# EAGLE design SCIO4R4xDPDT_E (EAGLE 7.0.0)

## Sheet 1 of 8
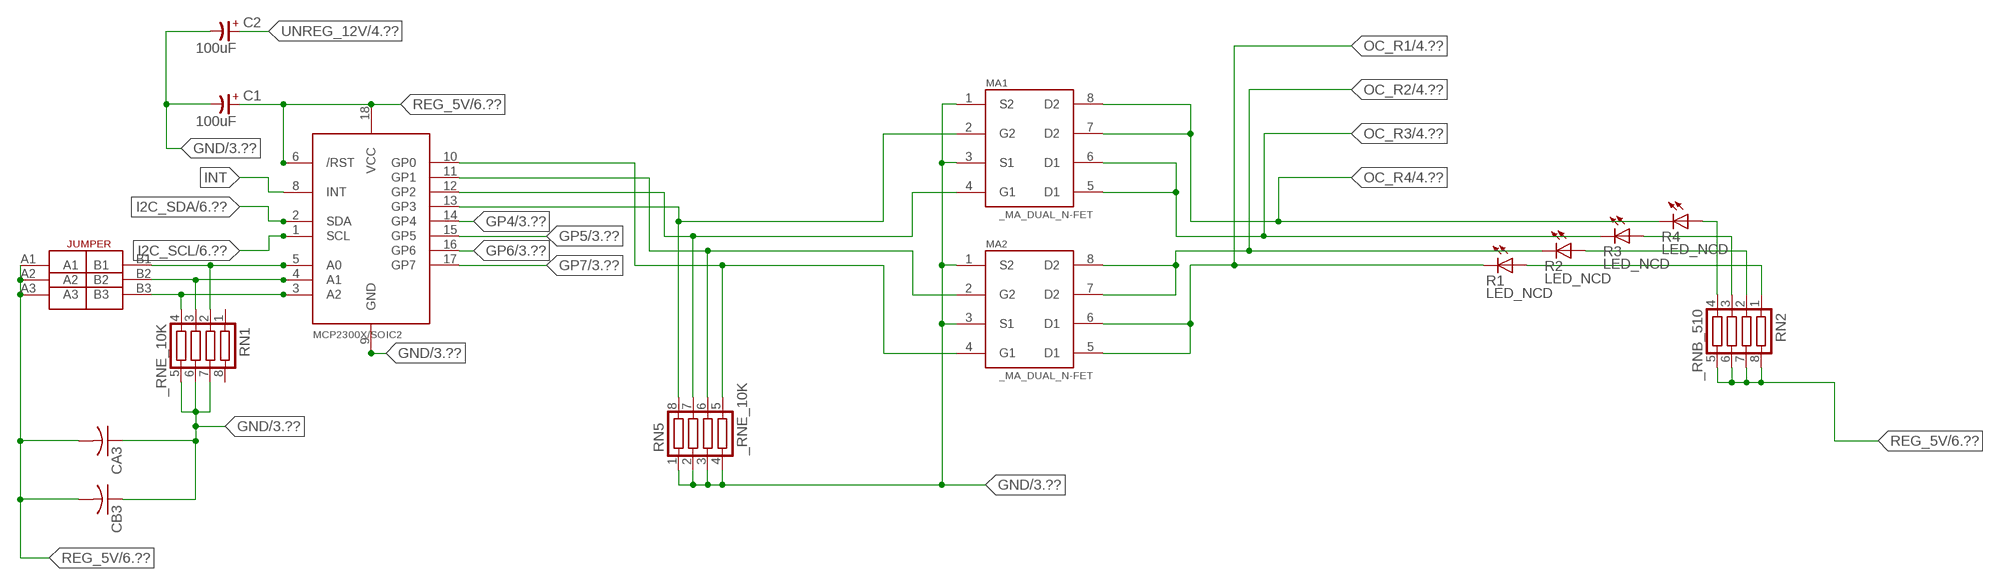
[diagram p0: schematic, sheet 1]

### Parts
C1  100uF  CP-E-025X060  [E-025X060]
C2  100uF  CP-E-025X060  [E-025X060]
CA3  CC1206KRX7R9BB104C1206K  [CC1206KRX7R9BB104]
CB3  TMK316F106ZL-TC1206K  [TMK316F106ZL-T]
IC2  MCP2300X/SO  [SO18W]
MA1  _MA_DUAL_N-FET  [_MA_DUAL_N-FET]
MA2  _MA_DUAL_N-FET  [_MA_DUAL_N-FET]
R1  LED_NCD  [CHIPLED_0603]
R2  LED_NCD  [CHIPLED_0603]
R3  LED_NCD  [CHIPLED_0603]
R4  LED_NCD  [CHIPLED_0603]
RN1  _RNE_10K  [RNE]
RN2  _RNB_510  [RNB]
RN5  _RNE_10K  [RNE]
U$18  JUMPER_3X2  [JUMPER_3X2]

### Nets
GND: C1.- C2.- CA3.1 CB3.1 IC2.9(GND) MA1.1(S2) MA1.3(S1) MA2.1(S2) MA2.3(S1) RN1.5 RN1.6 RN1.7 RN5.1 RN5.2 RN5.3 RN5.4 ; also sheet 3,6,8
GP4: IC2.14(GP4) ; also sheet 3
GP5: IC2.15(GP5) ; also sheet 3
GP6: IC2.16(GP6) ; also sheet 3
GP7: IC2.17(GP7) ; also sheet 3
I2C_SCL: IC2.1(SCL) ; also sheet 6
I2C_SDA: IC2.2(SDA) ; also sheet 6
INT: IC2.8(INT)
N$6: IC2.5(A0) RN1.2 U$18.B1
N$7: IC2.4(A1) RN1.3 U$18.B2
N$8: IC2.3(A2) RN1.4 U$18.B3
N$20: IC2.13(GP3) MA1.2(G2) RN5.8
N$21: IC2.12(GP2) MA1.4(G1) RN5.7
N$22: IC2.11(GP1) MA2.2(G2) RN5.6
N$23: IC2.10(GP0) MA2.4(G1) RN5.5
N$29: R4.A RN2.4
N$30: R3.A RN2.3
N$31: R2.A RN2.2
N$32: R1.A RN2.1
OC_R1: MA2.5(D1) MA2.6(D1) R1.C ; also sheet 4
OC_R2: MA2.7(D2) MA2.8(D2) R2.C ; also sheet 4
OC_R3: MA1.5(D1) MA1.6(D1) R3.C ; also sheet 4
OC_R4: MA1.7(D2) MA1.8(D2) R4.C ; also sheet 4
REG_5V: C1.+ CA3.2 CB3.2 IC2.6(/RST) IC2.18(VCC) RN2.5 RN2.6 RN2.7 RN2.8 U$18.A1 U$18.A2 U$18.A3 ; also sheet 6,8
UNREG_12V: C2.+ ; also sheet 4,6
Unconnected: RN1.1 RN1.8

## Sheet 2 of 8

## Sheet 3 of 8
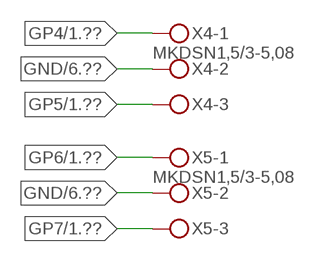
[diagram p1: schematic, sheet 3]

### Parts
X4  MKDSN1,5/3-5,08  [MKDSN1,5/3-5,08]
X5  MKDSN1,5/3-5,08  [MKDSN1,5/3-5,08]

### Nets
GND: X4.2 X5.2 ; also sheet 1,6,8
GP4: X4.1 ; also sheet 1
GP5: X4.3 ; also sheet 1
GP6: X5.1 ; also sheet 1
GP7: X5.3 ; also sheet 1

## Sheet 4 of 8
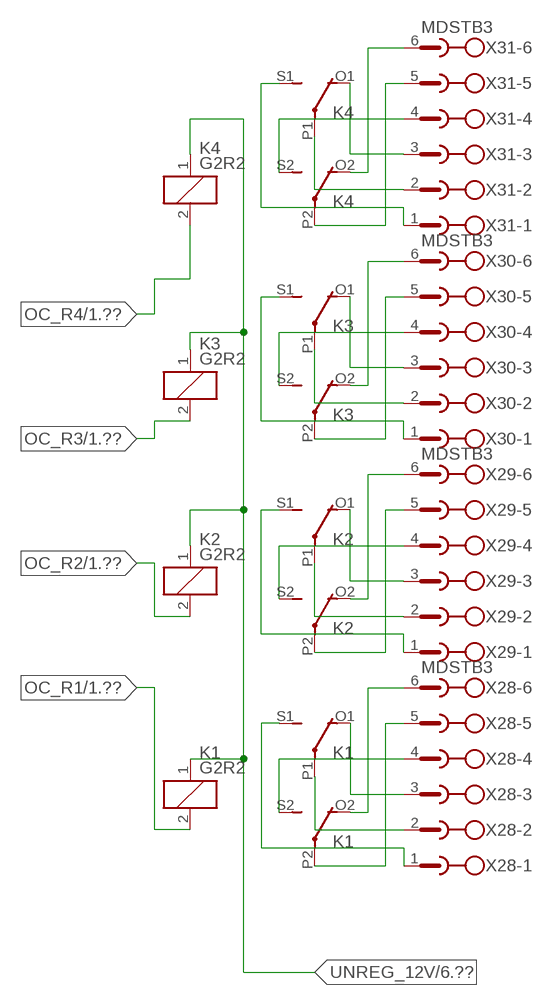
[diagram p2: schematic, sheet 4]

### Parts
K1  G2R2  [G2R2]
K2  G2R2  [G2R2]
K3  G2R2  [G2R2]
K4  G2R2  [G2R2]
X28  MDSTB3  [MDSTB3]
X29  MDSTB3  [MDSTB3]
X30  MDSTB3  [MDSTB3]
X31  MDSTB3  [MDSTB3]

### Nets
N$9: K3.P2(3:COM) X30.5
N$10: K3.O2(3:NC) X30.6
N$11: K4.P2(3:COM) X31.5
N$12: K4.O2(3:NC) X31.6
N$13: K3.S2(3:NO) X30.4
N$14: K4.S2(3:NO) X31.4
N$15: K3.O1(2:NC) X30.3
N$16: K4.O1(2:NC) X31.3
N$17: K4.P1(2:COM) X31.2
N$18: K3.P1(2:COM) X30.2
N$19: K3.S1(2:NO) X30.1
N$24: K4.S1(2:NO) X31.1
N$203: K1.P2(3:COM) X28.5
N$204: K1.O2(3:NC) X28.6
N$205: K1.S2(3:NO) X28.4
N$206: K1.P1(2:COM) X28.2
N$207: K1.O1(2:NC) X28.3
N$208: K1.S1(2:NO) X28.1
N$209: K2.P2(3:COM) X29.5
N$210: K2.O2(3:NC) X29.6
N$211: K2.S2(3:NO) X29.4
N$212: K2.S1(2:NO) X29.1
N$213: K2.P1(2:COM) X29.2
N$214: K2.O1(2:NC) X29.3
OC_R1: K1.2(1:C2) ; also sheet 1
OC_R2: K2.2(1:C2) ; also sheet 1
OC_R3: K3.2(1:C2) ; also sheet 1
OC_R4: K4.2(1:C2) ; also sheet 1
UNREG_12V: K1.1(1:C1) K2.1(1:C1) K3.1(1:C1) K4.1(1:C1) ; also sheet 1,6

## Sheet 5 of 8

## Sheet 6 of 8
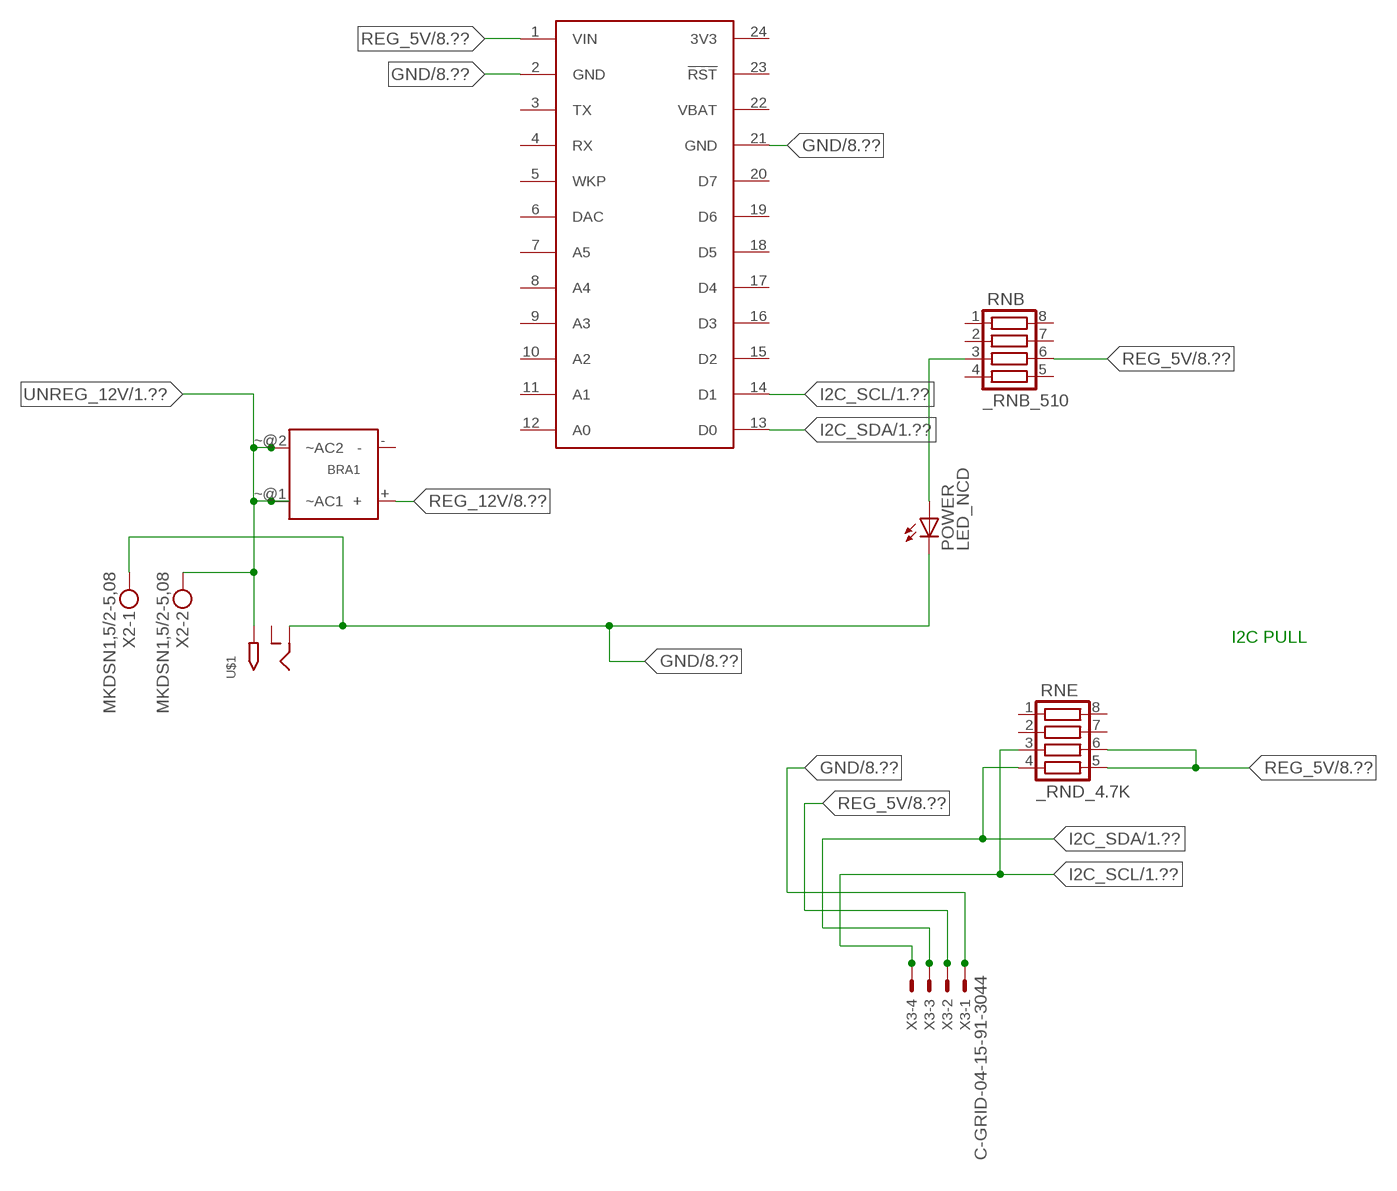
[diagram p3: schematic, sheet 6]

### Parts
BRA1  MB2S_  [MB2S]
POWER  LED_NCD  [CHIPLED_0603]
RNB  _RNB_510  [RNB]
RNE  _RND_4.7K  [RND]
S1  SPARK_CORECORE  [SPARK_CORE]
U$1  2.1MMJACK  [PJ-102A]
X2  MKDSN1,5/2-5,08  [MKDSN1,5/2-5,08]
X3  C-GRID-04-15-91-3044  [15-91-04]

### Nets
GND: POWER.C S1.2(GND) S1.21(GND) U$1.RING X2.1 X3.1 ; also sheet 1,3,8
I2C_SCL: RNE.3 S1.14(D1) X3.4 ; also sheet 1
I2C_SDA: RNE.4 S1.13(D0) X3.3 ; also sheet 1
N$2: POWER.A RNB.3
REG_5V: RNB.6 RNE.5 RNE.6 S1.1(VIN) X3.2 ; also sheet 1,8
REG_12V: BRA1.+ ; also sheet 8
UNREG_12V: BRA1.~@1(~AC1) BRA1.~@2(~AC2) U$1.TIP X2.2 ; also sheet 1,4
Unconnected: BRA1.- RNB.1 RNB.2 RNB.4 RNB.5 RNB.7 RNB.8 RNE.1 RNE.2 RNE.7 RNE.8 S1.3(TX) S1.4(RX) S1.5(WKP) S1.6(DAC) S1.7(A5) S1.8(A4) S1.9(A3) S1.10(A2) S1.11(A1) S1.12(A0) S1.15(D2) S1.16(D3) S1.17(D4) S1.18(D5) S1.19(D6) S1.20(D7) S1.23(!RST) U$1.RING_SW

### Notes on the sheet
- I2C PULL

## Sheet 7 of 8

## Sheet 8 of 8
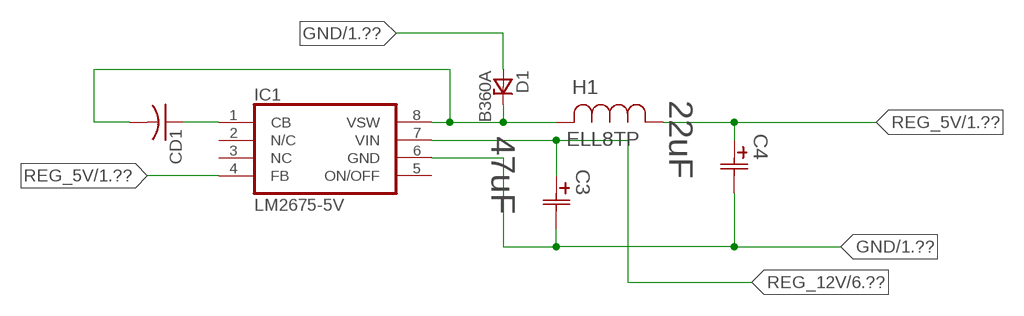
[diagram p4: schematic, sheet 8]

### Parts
C3  47uF  490-5463-6-NDCAP  [C2917(7343)-Y]
C4  22uF  490-5463-6-NDCAP  [C2917(7343)-Y]
CD1  _CD_10NF_50VC1206K  [_CD_10NF_50V]
D1  B360A  [DO214AC_ZENER]
H1  ELL8TP  [IND_ELL8TP]
IC1  LM2675-5V  LM2675  [SO-8]

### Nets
GND: C3.2(C2) C4.2(C2) D1.A IC1.6(GND) ; also sheet 1,3,6
N$1: CD1.2 D1.C H1.2 IC1.8(VSW)
N$3: CD1.1 IC1.1(CB)
REG_5V: C4.1(C1) H1.1 IC1.4(FB) ; also sheet 1,6
REG_12V: C3.1(C1) IC1.7(VIN) ; also sheet 6
Unconnected: IC1.2(N/C) IC1.5(ON/OFF)

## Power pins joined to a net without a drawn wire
3V3: S1.24(3V3)
NC: IC1.3(NC)
VBAT: S1.22(VBAT)

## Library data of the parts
BRA1 = NCD_ULTIMATE_LIBRARY:MB2S: Bridge Rectifier BRA MB2S 200V 500ma Digikey MB2S-TPMSTR-ND/MB2S-TP
C1 C2 = NCD_ULTIMATE_LIBRARY:CP-: Capacitors All Kinds POLARIZED CAP
C3 C4 = NCD_ULTIMATE_bhaskar:490-5463-6-ND: NCD CAP
CA3 = NCD_ULTIMATE_LIBRARY:CC1206KRX7R9BB104: Capacitor CA .1uF 50V SMT C1206K CC1206KRX7R9BB104
CB3 = NCD_ULTIMATE_LIBRARY:TMK316F106ZL-T: Capacitor CB 10uF SMT 1206 TMK316F106ZL-T
CD1 = NCD_ULTIMATE_LIBRARY:_CD_10NF_50V: Capacitor 10nF SMT
D1 = NCD_ULTIMATE_bhaskar:B360A: NCD DIODE B350A/B360A
H1 = NCD_ULTIMATE_bhaskar:ELL8TP: NCD coil
IC1 = NCD_ULTIMATE_bhaskar:LM2675: LM2675 NCD http://www.ti.com/lit/ds/symlink/lm2675.pdf
IC2 = NCD_ULTIMATE_LIBRARY:MCP2300X: Semiconductor Port Expander I/O 8-Bit I2C MCP23008 Inexpensive i2c i/o expander - 8 general purpose i/o pins with optional pullups
K1-K4 = NCD_ULTIMATE_LIBRARY:G2R2: RELAY 2 x switch, Omron
MA1 MA2 = NCD_ULTIMATE_LIBRARY:_MA_DUAL_N-FET: FET Dual N-Channel 8-SOIC NMOSFET Digikey 785-1064-2-ND/AO4842
POWER = NCD_ULTIMATE_bhaskar:LED_NCD
R1-R4 = NCD_ULTIMATE_LIBRARY:LED_NCD: LED Digikey 754-1132-2-ND/APT2012SRCPRV
RN1 RN5 = NCD_ULTIMATE_LIBRARY:_RNE_10K: Resistor Array RNE SMT 10K x 4 Single Resistor Source: http://www.ctscorp.com/components/Datasheets/CTSChipArrayDs.pdf Digikey 742C083103JPTR-ND/742C083103JP; OC_FARNELL: unknown; OC_NEWARK: unknown
RN2 RNB = NCD_ULTIMATE_LIBRARY:_RNB_510: Resistor Array RNB SMT 510 x 4 Single Resistor Source: http://www.ctscorp.com/components/Datasheets/CTSChipArrayDs.pdf Digikey 742C083511JPTR-ND/ 742C083511JP; OC_FARNELL: unknown; OC_NEWARK: unknown
RNE = NCD_ULTIMATE_LIBRARY:_RND_4.7K: Resistor Array RND SMT 4.7K x 4 Single Resistor Source: http://www.ctscorp.com/components/Datasheets/CTSChipArrayDs.pdf Digikey 742C083472JPTR-ND/742C083472JP; OC_FARNELL: unknown; OC_NEWARK: unknown
S1 = Spark:SPARK_CORE
U$1 = NCD_ULTIMATE_CONNECTORS:2.1MMJACK: 2.1mm x 5.5mm DC jack with internal switch. Digikey part #PJ-102A, 4UCON part #05537 By microbuilder.eu
U$18 = NCD_ULTIMATE_CONNECTORS:JUMPER_3X2
X2 = NCD_ULTIMATE_CONNECTORS:MKDSN1,5/2-5,08: MKDSN 1,5/ 2-5,08 Printklemme
X3 = NCD_ULTIMATE_CONNECTORS:C-GRID-04: CONNECTOR 4-Pos I2C wire to board 2.54 mm (0.100") pitch header Digikey WM1342-ND/0015912045; OC_FARNELL: unknown; OC_NEWARK: unknown
X4 X5 = NCD_ULTIMATE_CONNECTORS:MKDSN1,5/3-5,08: MKDSN 1,5/ 3-5,08 Printklemme Nennstrom: 13,5 A Nennspannung: 250 V Rastermaß: 5,08 mm Polzahl: 3 Anschlussart: Schraubanschluss Montage: Löten Anschlussrichtung Leiter/Platine: 0 ° Artikelnummer: 1729131 Source: http://eshop.phoenixcontact.com .. 1729131.pdf
X28-X31 = NCD_ULTIMATE_LIBRARY:MDSTB3: PHOENIX

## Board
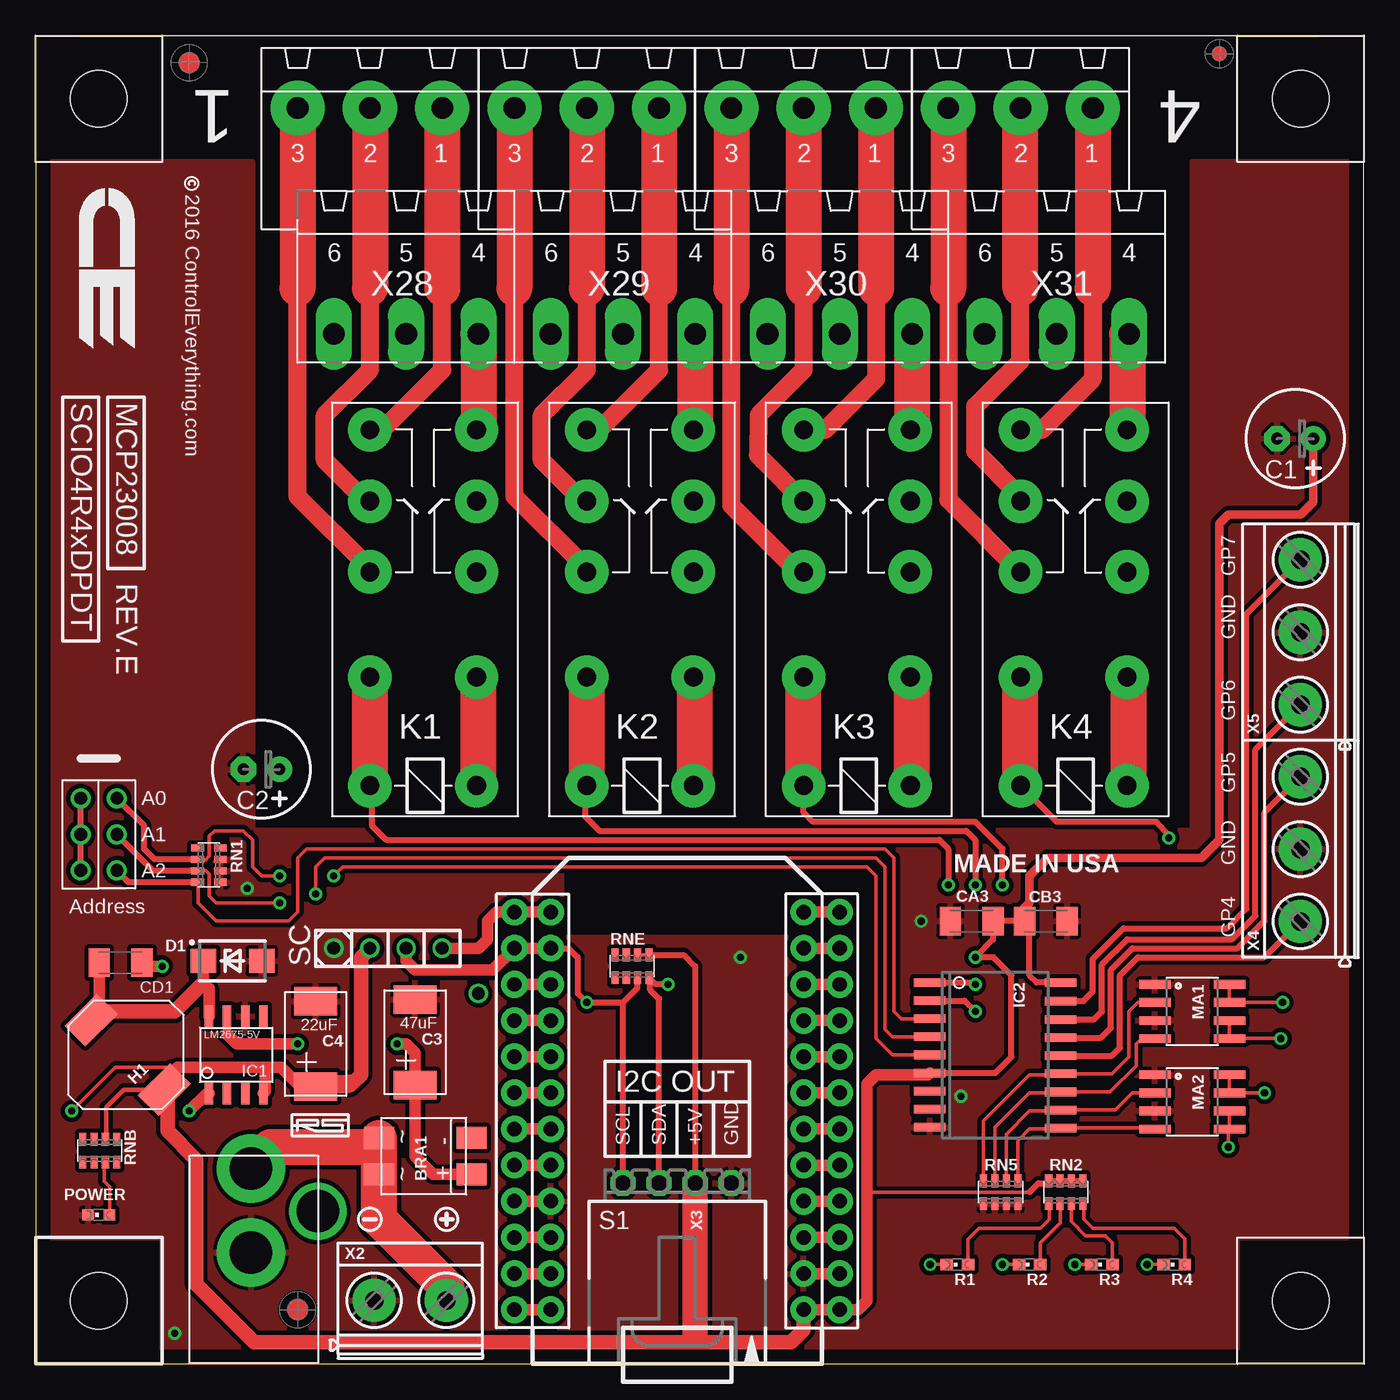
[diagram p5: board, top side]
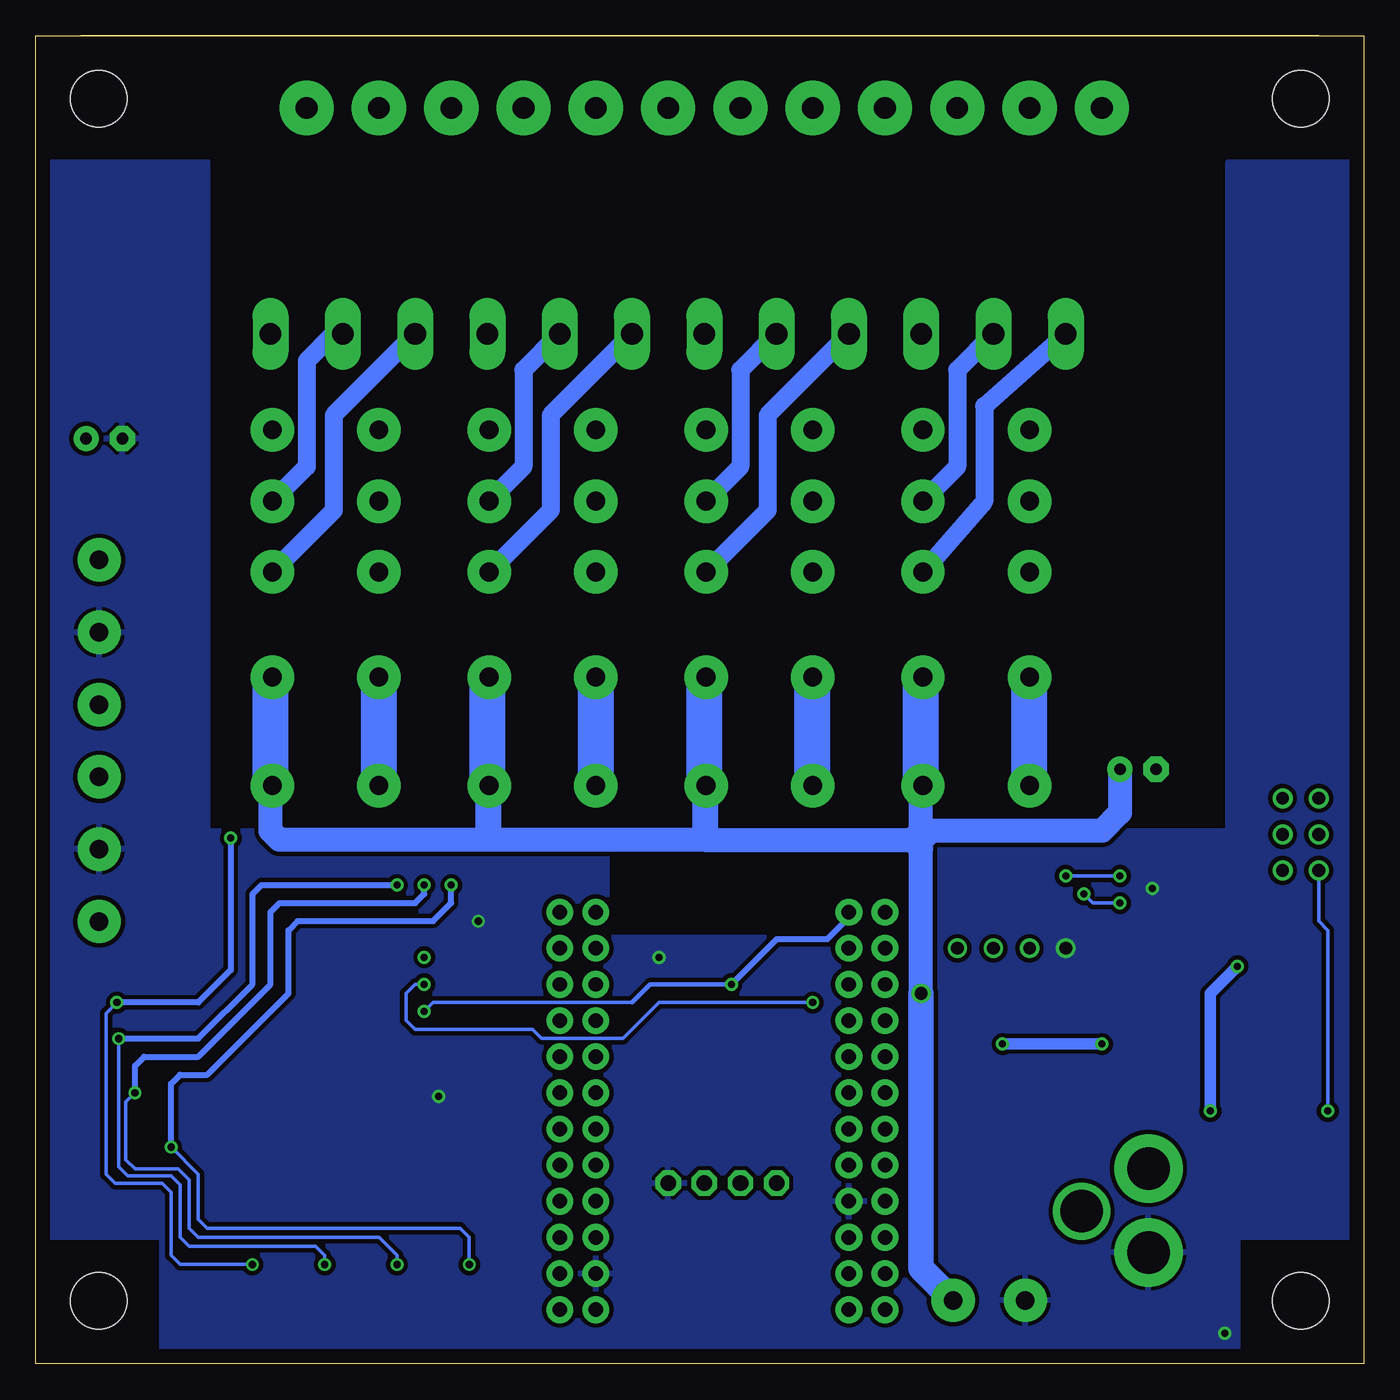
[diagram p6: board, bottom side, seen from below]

Size 93.34 x 93.34 mm. Coordinates in mm from the lower left corner, seen from the top.
Outline: 0,59.99 0,59.05
Outline: 0,59.05 0,0 79.38,0 93.34,0 93.34,93.34 0,93.34 0,59.05
Outline: 3.17,93.34 90.17,93.34
Copper layers (1*16): Top 0.035mm / dielectric 1.5mm / Bottom 0.035mm
Design rules "default": minimum track width 10mil, minimum drill 24mil, track to track 8mil, track to pad 8mil, pad to pad 8mil, via to via 8mil, smd to smd 8mil, copper to edge 40mil, drill to drill 8mil, minimum pad ring 10mil, minimum via ring 8mil, stop-mask expansion 4mil, vias tented up to drill 0mil, thermal gap 10mil
Holes 3.96 mm at 4.45,4.45

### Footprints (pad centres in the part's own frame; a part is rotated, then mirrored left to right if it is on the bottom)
MB2S = smd 1.55 x 2.1: + 0,-6.5; - 2.54,-6.5; ~@1 0,0; ~@2 2.54,0
E-025X060 = drill 0.813 pad 1.778: + -1.27,0 | drill 0.813 pad 1.778 octagon: - 1.27,0
C2917(7343)-Y = smd 2 x 3: 1 -3,0; 2 3,0
CC1206KRX7R9BB104 = smd 1.5 x 2: 1 -1.5,0; 2 1.5,0
TMK316F106ZL-T = smd 1.5 x 2: 1 -1.5,0; 2 1.5,0
_CD_10NF_50V = smd 1.5 x 2: 1 -1.5,0; 2 1.5,0
DO214AC_ZENER = smd 1.8 x 1.7: A 2.05,0; C -2.05,0
IND_ELL8TP = smd 2.054 x 3.2 rotated 45: 1 -2.442,-2.696; 2 2.442,2.442
SO-8 = smd 0.6 x 1.55: 1 -1.905,-2.69; 2 -0.635,-2.69; 3 0.635,-2.69; 4 1.905,-2.69; 5 1.905,2.71; 6 0.635,2.71; 7 -0.635,2.71; 8 -1.905,2.71
SO18W = smd 0.6 x 2.2: 1 -4.445,-4.6; 2 -3.175,-4.6; 3 -1.905,-4.6; 4 -0.635,-4.6; 5 0.635,-4.6; 6 1.905,-4.6; 7 3.175,-4.6; 8 4.445,-4.6; 9 5.715,-4.6; 10 5.775,4.6; 11 4.505,4.6; 12 3.235,4.6; 13 1.965,4.6; 14 0.695,4.6; 15 -0.575,4.6; 16 -1.845,4.6; 17 -3.145,4.6; 18 -4.445,4.6
G2R2 = drill 1.321 pad 3.048: 1 -2.54,-3.683; 2 -2.54,3.81; 3 5.08,-3.683; 4 5.08,3.81; O1 12.471,3.81; O2 12.471,-3.683; P1 17.45,3.81; P2 17.45,-3.683; S1 22.454,3.81; S2 22.454,-3.683
_MA_DUAL_N-FET = smd 0.61 x 2.21: 1 -1.905,-2.616; 2 -0.635,-2.616; 3 0.635,-2.616; 4 1.905,-2.616; 5 1.905,2.616; 6 0.635,2.616; 7 -0.635,2.616; 8 -1.905,2.616
CHIPLED_0603 = smd 0.8 x 0.8: A 0,-0.75; C 0,0.75
CHIPLED_0603' = smd 0.8 x 0.876: A 0,-0.75; C 0,0.75
RNE = smd 0.5 x 0.9: 1 -1.2,-0.8; 2 -0.4,-0.8; 3 0.4,-0.8; 4 1.2,-0.8; 5 1.2,0.8; 6 0.4,0.8; 7 -0.4,0.8; 8 -1.2,0.8
RNB = smd 0.5 x 0.9: 1 -1.2,-0.8; 2 -0.4,-0.8; 3 0.4,-0.8; 4 1.2,-0.8; 5 1.2,0.8; 6 0.4,0.8; 7 -0.4,0.8; 8 -1.2,0.8
RND = smd 0.5 x 0.9: 1 -1.2,-0.8; 2 -0.4,-0.8; 3 0.4,-0.8; 4 1.2,-0.8; 5 1.2,0.8; 6 0.4,0.8; 7 -0.4,0.8; 8 -1.2,0.8
SPARK_CORE = drill 1.016 pad 1.88: 1 -8.89,13.97; 2 -8.89,11.43; 3 -8.89,8.89; 4 -8.89,6.35; 5 -8.89,3.81; 6 -8.89,1.27; 7 -8.89,-1.27; 8 -8.89,-3.81; 9 -8.89,-6.35; 10 -8.89,-8.89; 11 -8.89,-11.43; 12 -8.89,-13.97; 13 8.89,-13.97; 14 8.89,-11.43; 15 8.89,-8.89; 16 8.89,-6.35; 17 8.89,-3.81; 18 8.89,-1.27; 19 8.89,1.27; 20 8.89,3.81; 21 8.89,6.35; 22 8.89,8.89; 23 8.89,11.43; 24 8.89,13.97; 25 -11.43,13.97; 26 -11.43,11.43; 27 -11.43,8.89; 28 -11.43,6.35; 29 -11.43,3.81; 30 -11.43,1.27; 31 -11.43,-1.27; 32 -11.43,-3.81; 33 -11.43,-6.35; 34 -11.43,-8.89; 35 -11.43,-11.43; 36 -11.43,-13.97; 37 11.43,13.97; 38 11.43,11.43; 39 11.43,8.89; 40 11.43,6.35; 41 11.43,3.81; 42 11.43,1.27; 43 11.43,-1.27; 44 11.43,-3.81; 45 11.43,-6.35; 46 11.43,-8.89; 47 11.43,-11.43; 48 11.43,-13.97
PJ-102A = drill 3 pad 4.8: RING 0.1,-3.39; TIP 0.1,-9.29 | drill 3 pad 3.251: RING_SW -4.6,-6.29
PCB_MOUNTING_HOLE = hole 3.962: 4.445,4.445
JUMPER_3X2 = drill 0.9: A1 0,5.08; A2 0,2.54; A3 0,0; B1 2.54,5.08; B2 2.54,2.54; B3 2.54,0
MKDSN1,5/2-5,08 = drill 1.3 pad 3.048: 1 -2.561,0.025; 2 2.519,0.025
15-91-04 = drill 1.1 pad 1.778 octagon: 1 -3.81,-7.62; 2 -1.27,-7.62; 3 1.27,-7.62; 4 3.81,-7.62
MKDSN1,5/3-5,08 = drill 1.3 pad 3.048: 1 -7.641,0.025; 2 -2.561,0.025; 3 2.519,0.025
MDSTB3 = drill 1.524 pad 3.81: 1 -3.81,-10.795; 2 1.27,-10.795; 3 6.35,-10.795 | drill 1.524 pad 2.54 long: 4 -6.35,5.08; 5 -1.27,5.08; 6 3.81,5.08

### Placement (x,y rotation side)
BRA1  24.13,13.34 90 top
C1  88.52,65.02 180 top
C2  15.88,41.78 180 top
C3  26.67,22.61 90 top
C4  19.68,22.48 90 top
CA3  65.79,31.12 0 top
CB3  70.99,31.12 180 top
CD1  5.97,28.19 180 top
D1  13.84,28.32 0 top
H1  6.35,21.72 90 top
IC1  14.1,21.72 0 top
IC2  67.44,22.35 270 top
K1  27.3,43.18 90 top
K2  42.55,43.18 90 top
K3  57.78,43.18 90 top
K4  73.03,43.18 90 top
MA1  81.28,24.77 270 top
MA2  81.28,18.41 270 top
POWER  4.45,10.48 90 top
R1  LED_NCD  [CHIPLED_0603']  64.77,6.98 90 top
R2  LED_NCD  [CHIPLED_0603']  69.85,6.98 90 top
R3  LED_NCD  [CHIPLED_0603']  74.93,6.98 90 top
R4  LED_NCD  [CHIPLED_0603']  80.01,6.98 90 top
RN1  12.19,35.05 270 top
RN2  72.39,12.07 0 top
RN5  67.82,12.07 0 top
RNB  4.51,14.99 0 top
RNE  41.91,27.94 0 top
S1  45.09,17.78 180 top
U$1  15.24,4.45 180 top
U$4  PCB_MOUNTING_HOLE  [PCB_MOUNTING_HOLE]  93.34,84.45 90 top
U$6  PCB_MOUNTING_HOLE  [PCB_MOUNTING_HOLE]  93.34,0 90 top
U$10  [VISION_REF15]  18.41,3.81 0 top
U$11  PCB_MOUNTING_HOLE  [PCB_MOUNTING_HOLE]  8.89,84.45 90 top
U$15  [VISION_REF15]  10.79,91.44 270 top
U$18  3.17,34.67 0 top
U$19  [VISION_REF10]  83.19,92.08 0 top
U$21  [ICON_USA]  64.52,34.54 0 top
U$22  [ICON_MINUS]  23.5,10.16 180 top
U$24  [ICON_PLUS]  28.89,10.16 90 top
X2  26.35,4.45 0 top
X3  45.09,5.08 180 top
X4  88.9,38.73 90 top
X5  88.9,53.97 90 top
X28  24.77,77.47 180 top
X29  40.01,77.47 180 top
X30  55.24,77.47 180 top
X31  70.48,77.47 180 top

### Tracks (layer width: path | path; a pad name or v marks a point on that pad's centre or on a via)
GND  (via drill 0.5, 0.9)
  other vias: 14.86,33.4 65.02,18.8 9.78,2.16 20.95,29.21 49.53,28.57 62.23,31.12
  pour Bottom (isolate 0.305): -3.81,8.89 8.89,8.89 8.89,0 84.45,0 84.45,8.89 92.71,8.89 92.71,84.45 81.28,84.45 81.28,37.46 9.53,37.46 9.53,84.45 -3.81,84.45
  pour Top (isolate 0.305): -8.26,8.89 8.89,8.89 8.89,0 84.45,0 84.45,8.89 92.71,8.89 92.71,84.45 81.28,84.45 81.28,37.46 15.24,37.46 15.24,84.45 -8.26,84.45
GP4
  Top 0.406: IC2.14 75.63,21.66 76.2,22.23 76.2,27.3 77.47,28.57 86.36,28.57 X4.1
GP5
  Top 0.406: IC2.15 74.87,22.93 75.56,23.62 75.56,27.69 77.09,29.21 84.45,29.21 86.36,31.12 86.36,38.74 X4.3
GP6
  Top 0.406: IC2.16 74.36,24.2 74.93,24.77 74.93,28.07 76.71,29.85 84.07,29.85 85.72,31.5 85.72,43.18 X5.1
GP7
  Top 0.406: IC2.17 73.63,25.5 74.3,26.16 74.3,28.45 76.45,30.61 83.69,30.61 85.09,32 85.09,52.71 X5.3
I2C_SCL  (via drill 0.5, 0.9)
  Top 0.406: IC2.1 65.91,26.8 v66.04,26.67 | X3.4 41.27,25.4 | 41.27,25.4 42.29,26.42 42.29,27.12 RNE.3 | S1.14 37.47,29.21 38.1,28.57 38.1,26.04 v38.73,25.4 41.27,25.4
  Top 0.813: v26.04,29.21 26.04,28.32 26.67,27.69 32.13,27.69 33.66,29.21
  Bottom 0.254: v38.73,25.4 49.53,25.4 52.07,22.86 57.78,22.86 58.42,23.5 66.67,23.5 67.31,24.13 67.31,26.04 66.67,26.67 v66.04,26.67
I2C_SDA  (via drill 0.5, 0.9)
  Top 0.406: IC2.2 65.28,25.53 v66.04,24.77 | X3.3 43.81,25.65 43.18,26.29 43.18,27.07 RNE.4 43.58,26.67 v44.45,26.67
  Top 0.813: v28.57,29.21 31.11,29.21 31.75,29.85 31.75,31.12 32.38,31.75 33.66,31.75
  Bottom 0.254: 51.44,25.4 65.41,25.4 v66.04,24.77
  Bottom 0.305: v44.45,26.67 50.16,26.67 51.44,25.4
  Bottom 0.406: S1.13 36.2,31.37 37.72,29.85 41.27,29.85 v44.45,26.67
N$1
  Top 0.813: H1.2 3.88,24.77 | D1.C 11.79,26.78 12.19,26.38 IC1.8 | CD1.2 4.47,24.79 4.45,24.77
  Top 1.016: 3.88,24.77 4.45,24.77 9.78,24.77 11.79,26.78
N$2
  Top 0.254: POWER.A 5.2,12.46 4.83,12.83 4.83,14.1 RNB.3
  Top 0.406: 4.95,14.14 RNB.3
N$3  (via drill 0.5)
  Top 0.813: IC1.1 12.04,19.03 v10.79,17.78 | v8.89,27.94 7.72,27.94 CD1.1
  Bottom 0.813: v10.79,17.78 10.79,26.04 v8.89,27.94
N$6  (via drill 0.5)
  Top 0.254: IC2.5 60.2,21.72 59.05,22.86 59.05,34.29 58.42,34.92 21.59,34.92 v20.95,34.29 | v17.14,34.29 15.88,34.29 15.24,34.92 15.24,36.83 14.61,37.46 12.57,37.46 12.19,37.08 12.19,35.69 11.94,35.43 11.41,35.43 RN1.2
  Top 0.406: RN1.2 8.36,35.45 7.62,36.2 7.62,37.85 U$18.B1
  Bottom 0.254: v20.95,34.29 v17.14,34.29
N$7  (via drill 0.5)
  Top 0.254: IC2.4 60.2,22.99 59.69,23.5 59.69,34.92 59.05,35.56 20.32,35.56 19.68,34.92 v19.68,33.02 | v17.14,32.38 12.7,32.38 12.19,32.89 12.19,34.42 11.94,34.67 11.41,34.67 RN1.3
  Top 0.406: RN1.3 8.27,34.65 U$18.B2
  Bottom 0.254: v19.68,33.02 19.05,32.38 v17.14,32.38
N$8
  Top 0.254: IC2.3 60.83,24.26 60.33,24.77 60.33,35.56 59.69,36.2 19.05,36.2 18.41,35.56 18.41,31.75 17.78,31.12 12.7,31.12 11.43,32.38 11.43,33.81 RN1.4
  Top 0.406: RN1.4 6.53,33.85 U$18.B3
N$9
  Bottom 1.27: X30.5 59.05,69.85 59.05,63.04 K3.P2
N$10
  Bottom 1.27: X30.6 57.15,66.67 57.15,59.97 K3.O2
N$11
  Bottom 1.27: X31.5 72.39,72.39 74.3,70.48 74.3,63.04 K4.P2
N$12
  Bottom 1.27: X31.6 72.39,66.67 72.39,59.97 K4.O2
N$13
  Top 2.54: X30.4 61.59,65.76 K3.S2
N$14
  Top 2.54: X31.4 76.71,72.39 K4.S2
N$15
  Top 1.27: K3.O1 53.57,55.65 48.9,60.32 48.9,75.56
  Top 2.54: X30.3 48.9,75.56
N$16
  Top 1.27: 64.14,75.56 64.14,60.73 K4.O1
  Top 2.54: X31.3 64.14,75.56
N$17
  Top 1.27: K4.P1 69.22,60.96 66.04,64.14 66.04,67.31 69.22,70.48 69.22,75.56
  Top 2.54: 69.22,75.56 X31.2
N$18
  Top 1.27: 53.98,75.56 53.98,69.85 50.8,66.67 50.75,63.88 51.1,63.5 K3.P1
  Top 2.54: X30.2 53.98,75.56
N$19
  Top 1.27: 59.05,75.56 59.05,69.22 55.47,65.63 K3.S1
  Top 2.54: X30.1 59.05,75.56
N$20
  Top 0.254: MA1.2 77.47,25.4 76.83,24.77 76.83,21.59 75.63,20.39 IC2.13 71.97,20.32 69.85,20.32 66.62,17.09 RN5.8
N$21
  Top 0.254: MA1.4 77.72,22.86 77.34,22.48 77.34,20.96 75.5,19.12 IC2.12 71.97,19.05 69.85,19.05 67.42,16.62 RN5.7
N$22
  Top 0.254: MA2.2 77.09,19.05 75.89,17.85 IC2.11 71.97,17.78 69.85,17.78 68.22,16.15 RN5.6
N$23
  Top 0.254: MA2.4 78.6,16.58 IC2.10 71.97,16.51 69.85,16.51 69.02,15.68 RN5.5
N$24
  Top 1.27: 74.3,75.56 74.3,69.22 70.71,65.63 K4.S1
  Top 2.54: X31.1 74.3,75.56
N$29
  Top 0.254: R4.A 80.76,8.77 80.01,9.52 74.3,9.52 73.66,10.16 73.66,11.2 RN2.4
N$30
  Top 0.254: R3.A 75.68,8.52 75.18,9.02 73.79,9.02 72.77,10.03 72.77,11.25 RN2.3
N$31
  Top 0.254: R2.A 70.6,8.5 72.01,9.91 72.01,11.25 RN2.2
N$32
  Top 0.254: R1.A 65.52,8.75 66.29,9.52 70.61,9.52 71.25,10.16 71.25,11.21 RN2.1
N$203
  Bottom 1.27: X28.5 28.57,69.85 28.57,63.04 K1.P2
N$204
  Bottom 1.27: X28.6 26.67,67.31 26.67,60.6 K1.O2
N$205
  Top 2.54: X28.4 31.11,65.76 K1.S2
N$206
  Top 1.27: K1.P1 23.19,60.63 20.32,63.5 20.32,66.67 23.5,69.85 23.5,75.56
  Top 2.54: X28.2 23.5,75.56
N$207
  Top 1.27: K1.O1 23.5,55.88 18.41,60.96 18.41,75.56
  Top 2.54: X28.3 18.41,75.56
N$208
  Top 1.27: K1.S1 24.36,65.63 28.57,69.85 28.57,75.56
  Top 2.54: X28.1 28.57,75.56
N$209
  Bottom 1.27: X29.5 43.81,69.85 43.81,63.04 K2.P2
N$210
  Bottom 1.27: X29.6 41.91,66.67 41.91,59.97 K2.O2
N$211
  Top 2.54: X29.4 46.35,65.76 K2.S2
N$212
  Top 1.27: K2.S1 39.37,65.41 43.81,69.85 43.81,75.56
  Top 2.54: X29.1 43.81,75.56
N$213
  Top 1.27: K2.P1 38.43,60.63 35.56,63.5 35.56,66.67 38.73,69.85 38.73,75.56
  Top 2.54: X29.2 38.73,75.56
N$214
  Top 1.27: K2.O1 38.73,55.88 33.66,60.96 33.66,75.56
  Top 2.54: X29.3 33.66,75.56
OC_R1  (via drill 0.5)
  Top 0.254: R1.C v62.87,6.98 | v83.82,15.24 83.82,16.43 MA2.5 MA2.6
  Top 0.406: v64.14,33.66 64.14,36.2 63.5,36.83 24.64,36.83 23.62,37.85 23.62,40.39 23.5,40.39 K1.2
  Bottom 0.254: v62.87,6.98 62.87,8.89 63.5,9.52 81.28,9.52 81.92,10.16 81.92,13.34 v83.82,15.24
  Bottom 0.406: v83.82,15.24 83.82,19.69 83.19,20.32 81.28,20.32 75.56,26.04 75.56,30.48 74.93,31.12 65.41,31.12 64.14,32.38 v64.14,33.66
OC_R2  (via drill 0.5)
  Top 0.254: R2.C v67.94,6.98 | v86.36,19.05 MA2.7 MA2.8
  Top 0.406: v66.04,33.66 66.04,36.83 65.41,37.46 39.62,37.46 38.61,38.48 38.61,40.64 K2.2
  Bottom 0.254: v67.94,6.98 67.94,7.62 69.22,8.89 81.92,8.89 82.55,9.52 82.55,12.95 83.31,13.72 86.36,13.72 87,14.35 87,18.41 v86.36,19.05
  Bottom 0.406: v86.36,19.05 86.36,20.96 85.72,21.59 81.92,21.59 76.83,26.67 76.83,31.75 76.2,32.38 66.67,32.38 66.04,33.02 v66.04,33.66
OC_R3  (via drill 0.5)
  Top 0.254: R3.C v73.03,6.98 | v87.5,22.86 MA1.5 MA1.6
  Top 0.406: v67.94,33.66 67.94,36.2 66.04,38.1 54.61,38.1 53.98,38.73 K3.2
  Bottom 0.254: v73.03,6.98 73.03,7.62 73.66,8.25 82.55,8.25 83.19,8.89 83.19,12.57 83.82,13.21 86.87,13.21 87.5,13.84 v87.5,22.86
  Bottom 0.406: v87.5,22.86 81.92,22.86 78.11,26.67 78.11,33.02 77.47,33.66 v67.94,33.66
OC_R4  (via drill 0.5)
  Top 0.254: R4.C v78.11,6.98 | v87.63,25.4 MA1.7 MA1.8
  Top 0.406: v79.63,36.96 79.63,37.08 78.74,38.1 71.75,38.1 K4.2
  Bottom 0.254: v78.11,6.98 83.19,6.98 83.82,7.62 83.82,12.07 84.45,12.7 87.76,12.7 88.39,13.34 88.39,24.64 v87.63,25.4
  Bottom 0.406: v79.63,36.96 79.63,27.69 81.92,25.4 v87.63,25.4
REG_5V  (via drill 0.5, 0.9)
  Top 0.229: 58.42,12.07 69.85,12.07
  Top 0.254: RNE.6 RNE.5 | 9.96,20.83 5.59,20.83 v2.54,17.78
  Top 0.305: 62.71,20.32 60.96,20.32 | H1.1 6.19,19.28 4.95,18.03 4.95,15.83 RNB.6
  Top 0.406: U$18.A3 U$18.A2 U$18.A1 | IC2.18 70.36,26.8 69.85,27.3 69.85,30.76 CB3.2 CA3.2 67.29,29.82 v66.04,28.57 67.31,28.57 68.58,27.3 68.58,21.59 67.44,20.45 IC2.6 | 69.85,12.07 70.48,12.7 71.03,12.7 RN2.8 RN2.7 RN2.6 RN2.5 | RNE.5 45.55,28.74 46.35,27.94 X3.2
  Top 0.61: C1.+ 89.79,60.58 88.9,59.69 83.82,59.69 83.19,59.05 83.19,36.83 81.92,35.56 71.12,35.56 69.85,34.29 69.85,32.38 69.22,31.75 69.22,31.39 CB3.2
  Top 0.813: 16.13,20.83 9.96,20.83 H1.1 | 16.13,20.83 17.27,20.83 18.41,19.69 20.75,19.69 C4.1 | IC1.4 16.13,19.15 16.13,20.83 | 56.52,3.81 57.78,3.81 58.42,4.45 58.42,12.07 58.42,19.69 59.05,20.32 62.71,20.32 IC2.6
  Top 1.016: 46.35,2.16 46.35,1.52 | 46.35,1.52 15.37,1.52 11.3,5.59 11.3,14.35 9.27,16.38 9.27,18.41 H1.1 | 22.05,19.69 22.23,19.69 22.86,20.32 22.86,28.57 v23.5,29.21 | S1.1 53.98,2.41 53.09,1.52 46.35,1.52
  Top 1.27: 20.75,19.69 22.05,19.69
  Top 1.778: X3.2 46.35,2.16
  Bottom 0.254: v2.54,17.78 2.54,30.48 3.17,31.12 U$18.A3
REG_12V  (via drill 0.5)
  Top 0.61: IC1.7 13.46,23.16 | 14.1,22.48 14.15,22.48
  Top 0.813: v18.41,22.48 14.15,22.48 13.46,23.16 | v25.4,22.48 26.04,22.48 26.67,21.84 C3.1 26.67,14.61 27.94,13.34 BRA1.+
  Bottom 0.813: v18.41,22.48 v25.4,22.48
UNREG_12V  (via drill 0.9)
  Top 2.54: X2.2 28.87,5.42 24.13,10.16 BRA1.~@1 24.13,15.24 | 24.13,15.24 BRA1.~@2 | U$1.TIP 15.14,13.87 16.51,15.24 24.13,15.24
  Bottom 1.676: 45.72,36.83 31.75,36.83 | 31.75,36.83 31.11,37.46 31.11,40.51 K1.1 | 45.72,36.83 46.35,37.46 46.35,40.51 K2.1 46.23,36.96 46.35,36.83 | 46.35,36.83 45.72,36.83 | 46.35,36.83 60.96,36.83 | 61.47,37.34 61.59,37.46 61.59,40.51 K3.1 61.47,37.34 | 61.47,37.34 60.96,36.83 | 60.96,36.83 76.2,36.83 76.83,37.46 76.83,40.51 K4.1 | v31.11,26.04 31.11,36.2 31.43,36.51 | 31.43,36.51 31.75,36.83 | C2.+ 17.14,38.73 18.41,37.46 30.48,37.46 31.43,36.51
  Bottom 1.778: v31.11,26.04 31.11,6.71 X2.2

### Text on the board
tNames: 1 | 4 | 2016 ControlEverything.com | SCIO4R4xDPDT | MCP23008 | REV.E | GP7 | GND | GP6 | GP5 | A0 | A1 | GND | A2 | Address | GP4 | SC | I2C OUT | SCL | SDA | +5V | GND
